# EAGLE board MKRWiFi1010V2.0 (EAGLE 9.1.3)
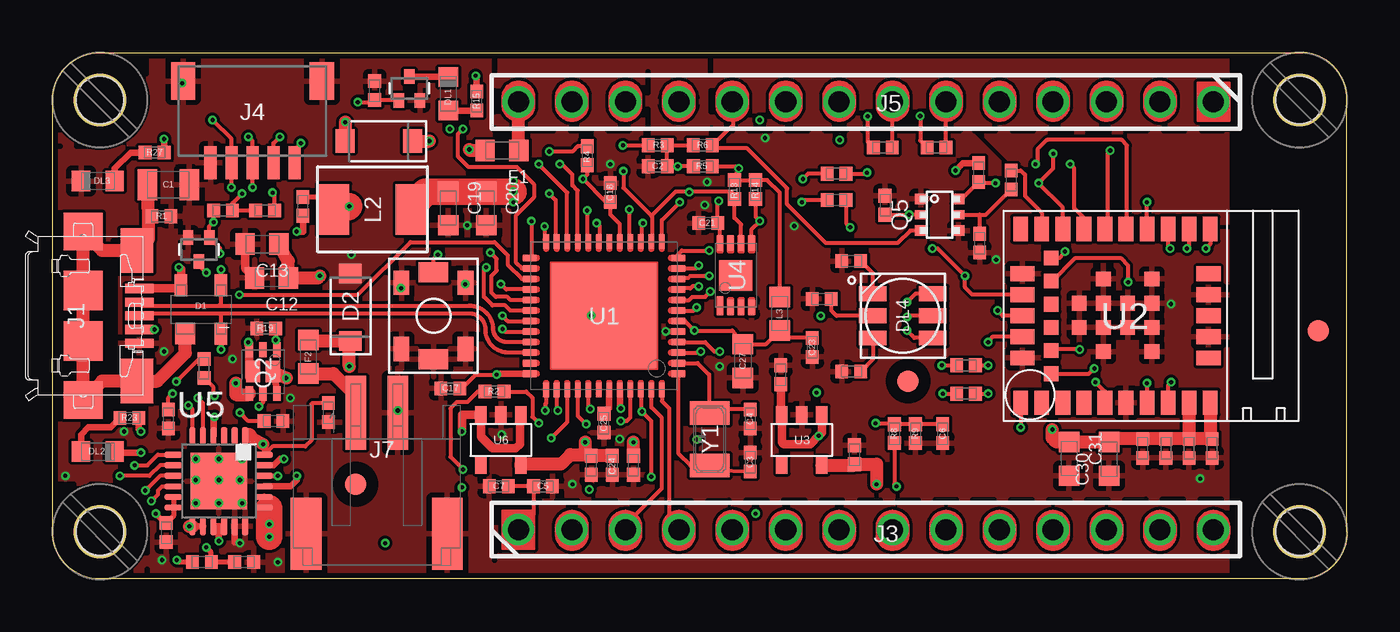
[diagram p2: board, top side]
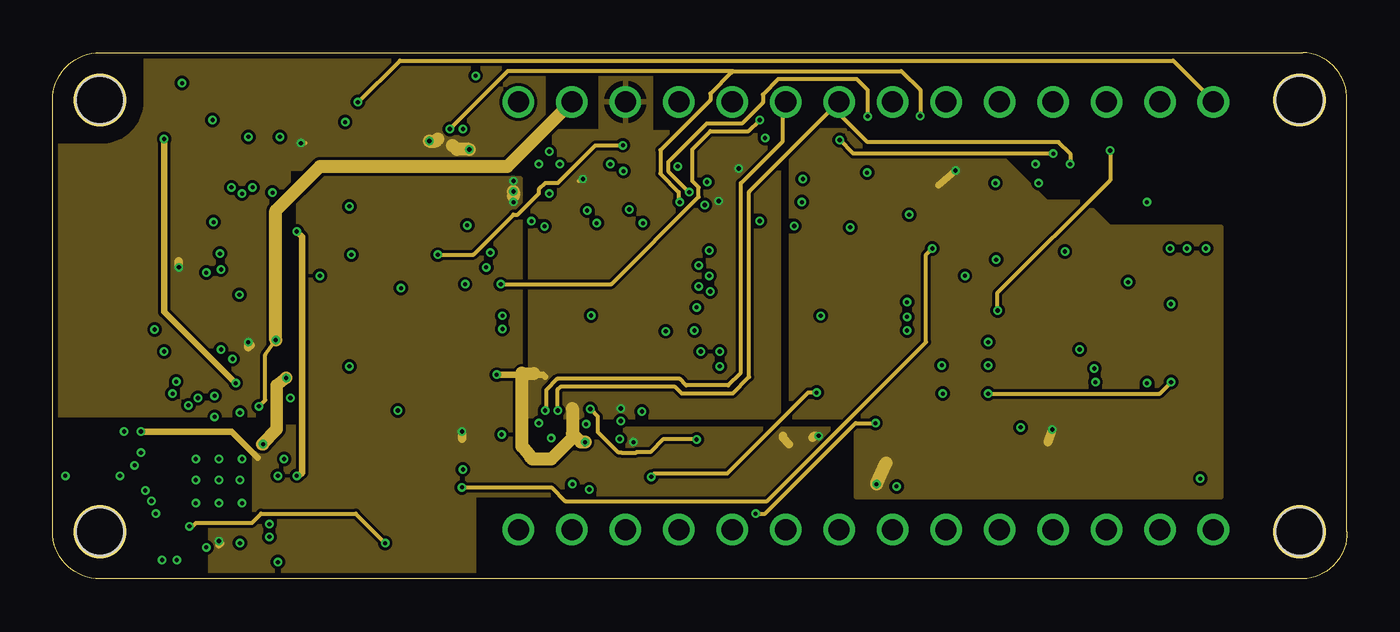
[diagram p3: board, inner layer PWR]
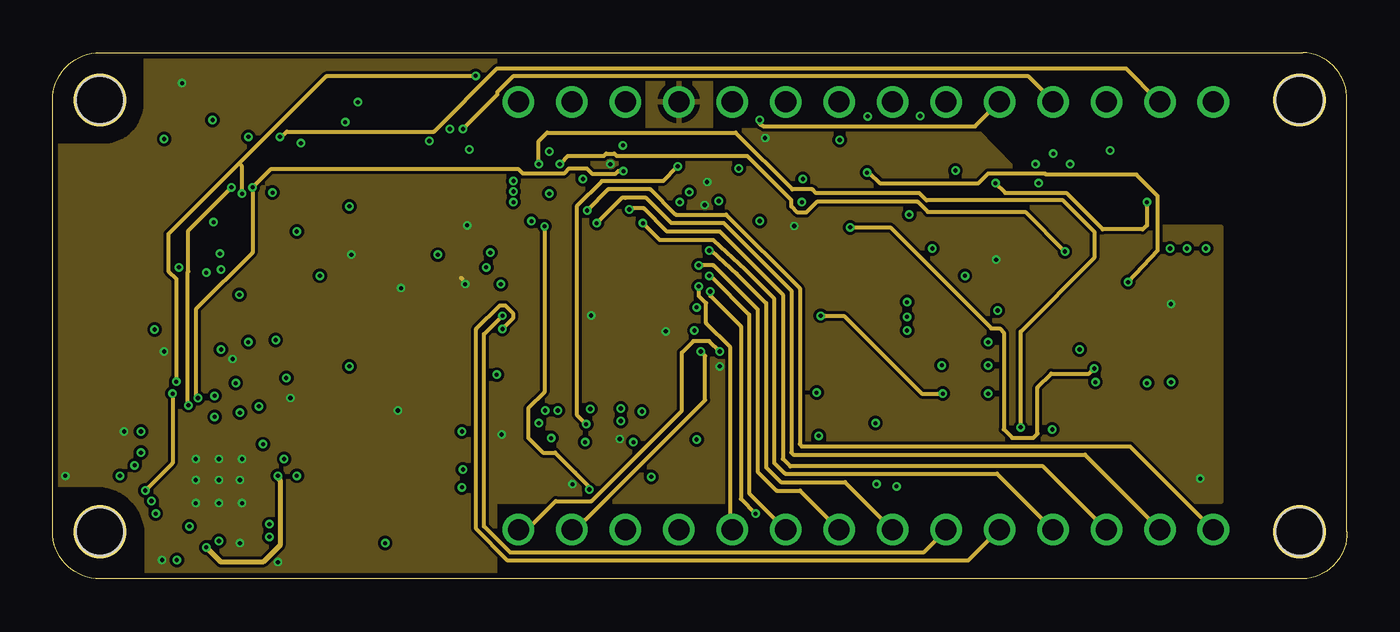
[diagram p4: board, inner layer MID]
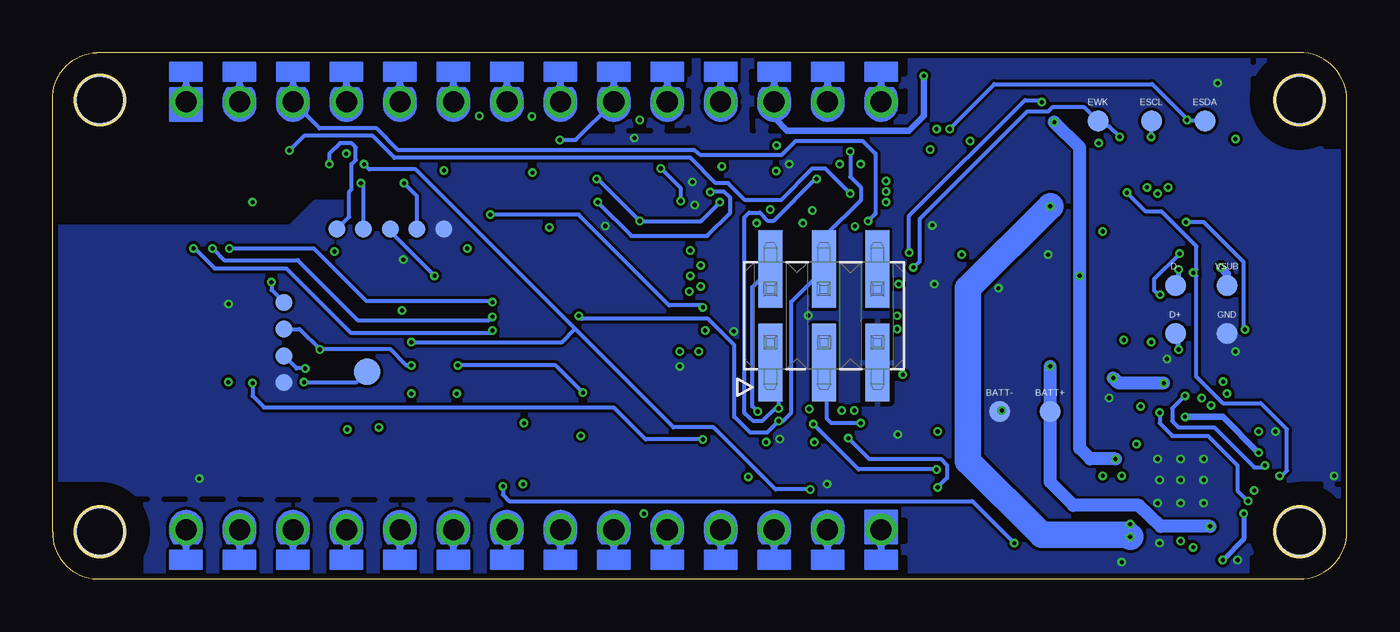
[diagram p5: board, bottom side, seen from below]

Size 61.5 x 25 mm. Coordinates in mm from the lower left corner, seen from the top.
Outline: 0,2.25 0,22.75 arc-90 2.25,25 59.4,25 arc-90 61.5,22.75 61.5,2.25 arc-90 59.4,0 2.25,0 arc-90 0,2.25
Copper layers (1*2*15*16): Top 0.035mm / dielectric 0.2mm / PWR 0.0175mm / dielectric 0.3mm / MID 0.0175mm / dielectric 0.2mm / Bottom 0.035mm
Design rules "B&B_4layers *": minimum track width 6mil, minimum drill 0.195mm, track to track 5.5mil, track to pad 5.5mil, pad to pad 5mil, via to via 5mil, smd to smd 0mil, copper to edge 10mil, drill to drill 8mil, minimum pad ring 6mil, minimum via ring 4mil, stop-mask expansion 4mil, vias tented up to drill 25mil, thermal gap 10mil
Net classes: 0 default: width 0.19 mm, drill 0.19 mm; 1 usb: width 0.19 mm, drill 0.19 mm, clearance 0.127 mm
Holes 2.25 mm at 2.25,2.25 59.25,2.25 59.25,22.75 2.25,22.75
tRestrict: area 0,0 to 4.5,4.5; area 0,20.5 to 4.5,25; area 57,20.5 to 61.5,25; area 57,0 to 61.5,4.5; 119 lines
bRestrict: area 0,0 to 4.5,4.5; area 0,20.5 to 4.5,25; area 57,0 to 61.5,4.5; area 57,20.5 to 61.5,25; 119 lines

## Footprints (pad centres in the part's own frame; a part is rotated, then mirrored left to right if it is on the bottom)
TP-1.00MM = smd 1 x 1 bottom: X 0,0
0805-R2013X50N = smd 0.95 x 1.45: 1 -1,0; 2 1,0
0402-1005X55N = smd 0.62 x 0.62: 1 -0.45,0; 2 0.45,0
0603-1608X90N = smd 0.95 x 1: 1 -0.8,0; 2 0.8,0
SOT190P230X110-4N = smd 1 x 1: 1 -1.15,0.75 | smd 1 x 0.6: 2 -1.15,-0.95; 3 1.15,-0.95; 4 1.15,0.95
SODFL3517X110N = smd 0.91 x 1.07: A 1.605,0; C -1.605,0
LEDC1608X80N-AK = smd 0.9 x 0.95: A 0.8,0; C -0.8,0
RGBLED = smd 1.3 x 0.7: 1 -1.425,1.05; 2 -1.425,0; 3 -1.425,-1.05; 4 1.425,-1.05; 5 1.425,0; 6 1.425,1.05
FD-1-1.5 = smd 1.016 x 1.016: P$1 0,0
TP-0.8MM = smd 0.8 x 0.8 bottom: X 0,0
ZX62-AB-5PA = smd 0.4 x 1.35: 1 -1.3,3.025; 2 -0.65,3.025; 3 0,3.025; 4 0.65,3.025; 5 1.3,3.025 | smd 2.1 x 1.6: 6 3.1,2.9; 11 -3.1,2.9 | smd 1.8 x 1.9: 7 4,0.35; 10 -4,0.35 | smd 1.9 x 1.9: 8 1.2,0.35; 9 -1.2,0.35
2X3_SMT = smd 1.143 x 3.683: 1 -2.54,-2.223; 2 -2.54,2.223; 3 0,-2.223; 4 0,2.223; 5 2.54,-2.223; 6 2.54,2.223
1X14_SMD_TH = drill 1: 1 0,0; 2 2.54,0; 3 5.08,0; 4 7.62,0; 5 10.16,0; 6 12.7,0; 7 15.24,0; 8 17.78,0; 9 20.32,0; 10 22.86,0; 11 25.4,0; 12 27.94,0; 13 30.48,0; 14 33.02,0
SM05B-SRSS-TB = smd 0.6 x 1.55: 1 -2,2.425; 2 -1,2.425; 3 0,2.425; 4 1,2.425; 5 2,2.425 | smd 1.2 x 1.8: SH1 -3.3,-1.45; SH2 3.3,-1.45
JST-S2B-PH-SM4-TB = smd 1 x 3.5: 1 -1,2.95; 2 1,2.95 | smd 1.5 x 3.4: 3 3.35,-2.8; 4 -3.35,-2.8
SRP4020 = smd 1.5 x 2.4: 1 -1.85,0; 2 1.85,0
TP-1.27MM = smd 1.27 x 1.27 bottom: X 0,0
C&K_PTS820_NO_HOLES = smd 1.15 x 0.75: 1 -1.575,1.525; 2 -1.575,-1.525; 3 1.575,1.525; 4 1.575,-1.525 | smd 0.95 x 1.4: 5 -2.075,0; 6 2.075,0
SOTFL50P160X78-3 = smd 0.5 x 0.66: D 0,0.57; G -0.5,-0.57; S 0.5,-0.57
SON65P205X205X75-8N-MWSD = smd 0.67 x 0.37: A 1.04,-0.65; D 1.04,0.65; G -1.04,0; K -1.04,-0.65; NC 1.04,0; S -1.04,0.65 | smd 1 x 0.7: D2 0,0.467; K2 0,-0.467
SOT363 = smd 0.6 x 0.5: 1 -0.9,0.75; 3 -0.9,-0.75; 4 0.9,-0.75; 6 0.9,0.75 | smd 0.6 x 0.4: 2 -0.9,0; 5 0.9,0
QFN50P700X700X90-49XN-EPSQ515 = smd 0.65 x 0.28: 1 -3.525,2.75; 2 -3.525,2.25; 3 -3.525,1.75; 4 -3.525,1.25; 5 -3.525,0.75; 6 -3.525,0.25; 7 -3.525,-0.25; 8 -3.525,-0.75; 9 -3.525,-1.25; 10 -3.525,-1.75; 11 -3.525,-2.25; 12 -3.525,-2.75; 25 3.525,-2.75; 26 3.525,-2.25; 27 3.525,-1.75; 28 3.525,-1.25; 29 3.525,-0.75; 30 3.525,-0.25; 31 3.525,0.25; 32 3.525,0.75; 33 3.525,1.25; 34 3.525,1.75; 35 3.525,2.25; 36 3.525,2.75 | smd 0.28 x 0.65: 13 -2.75,-3.525; 14 -2.25,-3.525; 15 -1.75,-3.525; 16 -1.25,-3.525; 17 -0.75,-3.525; 18 -0.25,-3.525; 19 0.25,-3.525; 20 0.75,-3.525; 21 1.25,-3.525; 22 1.75,-3.525; 23 2.25,-3.525; 24 2.75,-3.525; 37 2.75,3.525; 38 2.25,3.525; 39 1.75,3.525; 40 1.25,3.525; 41 0.75,3.525; 42 0.25,3.525; 43 -0.25,3.525; 44 -0.75,3.525; 45 -1.25,3.525; 46 -1.75,3.525; 47 -2.25,3.525; 48 -2.75,3.525 | smd 5 x 5: 49 0,0
NINA-W1X = smd 0.7 x 1.15: 1 4.95,4.125; 2 3.95,4.125; 3 2.95,4.125; 4 1.95,4.125; 5 0.95,4.125; 6 -0.05,4.125; 7 -1.05,4.125; 8 -2.05,4.125; 9 -3.05,4.125; 10 -4.05,4.125; 16 -4.05,-4.125; 17 -3.05,-4.125; 18 -2.05,-4.125; 19 -1.05,-4.125; 20 -0.05,-4.125; 21 0.95,-4.125; 22 1.95,-4.125; 23 2.95,-4.125; 24 3.95,-4.125; 25 4.95,-4.125 | smd 1.15 x 0.7: 11 -3.975,2; 12 -3.975,1; 13 -3.975,0; 14 -3.975,-1; 15 -3.975,-2; 26 4.875,-2; 27 4.875,-1; 28 4.875,0; 29 4.875,1; 30 4.875,2 | smd 0.7 x 0.7: 31 3.5,2.75; 32 3.5,1.65; 33 3.5,0.55; 34 3.5,-0.55; 35 3.5,-1.65; 36 3.5,-2.75; GND@1 -1.28,1.7; GND@2 -1.28,0.55; GND@3 -1.28,-0.6; GND@4 -1.28,-1.75; GND@5 -0.13,0.55; GND@6 -0.13,-0.6; GND@7 1.02,1.7; GND@8 1.02,0.55; GND@9 1.02,-0.6; GND@10 1.02,-1.75; GND@11 2.17,0.55; GND@12 2.17,-0.6
SOT25 = smd 0.55 x 0.8: 1 0.95,1.2; 2 0,1.2; 3 -0.95,1.2; 4 -0.95,-1.2; 5 0.95,-1.2
SON50P300X200X60-9N-EP160X140 = smd 0.85 x 0.3: 1 -1.45,0.75 | smd 0.7 x 0.3: 2 -1.525,0.25; 3 -1.525,-0.25; 4 -1.525,-0.75; 5 1.525,-0.75; 6 1.525,-0.25; 7 1.525,0.25; 8 1.525,0.75 | smd 1.4 x 1.6: 9 0,0
QFN24 = smd 0.3 x 0.85: 1 1.25,2.155; 2 0.75,2.155; 3 0.25,2.155; 4 -0.25,2.155; 5 -0.75,2.155; 6 -1.25,2.155; 13 -1.25,-2.155; 14 -0.75,-2.155; 15 -0.25,-2.155; 16 0.25,-2.155; 17 0.75,-2.155; 18 1.25,-2.155 | smd 0.85 x 0.3: 7 -2.155,1.25; 8 -2.155,0.75; 9 -2.155,0.25; 10 -2.155,-0.25; 11 -2.155,-0.75; 12 -2.155,-1.25; 19 2.155,-1.25; 20 2.155,-0.75; 21 2.155,-0.25; 22 2.155,0.25; 23 2.155,0.75; 24 2.155,1.25 | smd 2.7 x 2.7: 25 0,0
ABS07 = smd 1.1 x 1.9: 1 -1.25,0; 2 1.25,0

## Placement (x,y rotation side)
BATT+  DNP  [TP-1.00MM]  14.1,7.95 0 top
BATT-  DNP  [TP-1.00MM]  16.5,7.95 0 top
C1  4n7  [0805-R2013X50N]  5.5,18.73 0 top
C2  100n  [0402-1005X55N]  28.75,19.6 180 top
C3  20p  [0402-1005X55N]  33.15,5.55 270 top
C4  20p  [0402-1005X55N]  33.15,7.6 90 top
C5  4u7  [0402-1005X55N]  23.3,4.4 0 top
C6  100n  [0402-1005X55N]  42.3,6.9 270 top
C7  100n  [0402-1005X55N]  21.2,4.4 180 top
C8  100n  [0402-1005X55N]  55.1,6.2 270 top
C9  100n  [0402-1005X55N]  54,6.2 90 top
C12  10u  [0603-1608X90N]  10.4,14.3 180 top
C13  10u  [0603-1608X90N]  9.95,15.9 180 top
C14  1u  [0402-1005X55N]  13.1,7.9 270 top
C15  47n  [0402-1005X55N]  11.9,17.7 90 top
C16  4u7  [0402-1005X55N]  9.1,0.8 0 top
C17  100n  [0402-1005X55N]  18.9,9.05 180 top
C18  100n  [0402-1005X55N]  26.5,18.35 90 top
C19  10u  [0603-1608X90N]  18.8,17.6 270 top
C20  10u  [0603-1608X90N]  20.6,17.6 270 top
C21  100n  [0402-1005X55N]  31.15,16.9 180 top
C22  1u  [0402-1005X55N]  27.6,5.4 270 top
C23  100n  [0402-1005X55N]  36.1,11 270 top
C24  100n  [0402-1005X55N]  26.6,5.4 270 top
C25  1u  [0402-1005X55N]  26.2,7.4 270 top
C26  1u  [0402-1005X55N]  25.6,5.4 270 top
C27  4u7  [0603-1608X90N]  32.8,10.35 270 top
C28  DNP  [0402-1005X55N]  52.9,6.2 90 top
C29  DNP  [0402-1005X55N]  51.8,6.2 270 top
C30  DNP  [0603-1608X90N]  50.2,5.7 90 top
C31  DNP  [0603-1608X90N]  48.3,5.7 270 top
C32  1u  [0402-1005X55N]  34.6,9.7 90 top
C33  1u  [0402-1005X55N]  38.1,5.9 90 top
D1  PRTR5V  [SOT190P230X110-4N]  7.05,12.8 90 top
D2  PMEG6020  [SODFL3517X110N]  14.15,12.9 90 top
D3  PMEG6020  [SODFL3517X110N]  15.5,20.8 180 top
D+  DNP  [TP-1.00MM]  8.15,11.65 0 top
D-  DNP  [TP-1.00MM]  8.15,13.95 0 top
DL1  YELLOW  [LEDC1608X80N-AK]  18.8,23.05 270 top
DL2  ORANGE  [LEDC1608X80N-AK]  2.15,6.05 180 top
DL3  GREEN  [LEDC1608X80N-AK]  2.15,18.9 0 top
DL4  RGB  [RGBLED]  40.4,12.5 180 top
ESCL  DNP  [TP-1.00MM]  9.29,21.75 0 top
ESDA  DNP  [TP-1.00MM]  6.75,21.75 0 top
EWK  DNP  [TP-1.00MM]  11.83,21.75 0 top
F1  MFFSMF050  [0603-1608X90N]  21.35,20.35 180 top
F2  MFFSMF050  [0603-1608X90N]  12.15,10.55 90 top
FD1  DNP  [FD-1-1.5]  14.4,4.5 0 top
FD2  DNP  [FD-1-1.5]  60.15,11.8 0 top
FD3  DNP  [FD-1-1.5]  40.65,9.4 0 top
FRAME1  DNP  [FRAME]  not placed on the board
FRAME2  [FRAME-NO-BAN-FRAMEONLY]  not placed on the board
GND  DNP  [TP-1.00MM]  5.7,11.65 0 top
GPIO0  DNP  [TP-0.8MM]  45.46,16.62 0 top
J1  -  [ZX62-AB-5PA]  1.1,12.5 270 top
J2  DNP  [2X3_SMT]  24.85,12.5 0 bottom
J3  -  [1X14_SMD_TH]  22.13,2.34 0 top
J4  -  [SM05B-SRSS-TB]  9.5,22.2 180 top
J5  -  [1X14_SMD_TH]  55.15,22.66 180 top
J7  -  [JST-S2B-PH-SM4-TB]  15.4,4.95 0 top
JCLK  DNP  [TP-0.8MM]  50.5,13.13 0 top
JGND  DNP  [TP-0.8MM]  50.5,9.32 0 top
JTDO  DNP  [TP-0.8MM]  50.5,11.87 0 top
JTMS  DNP  [TP-0.8MM]  50.5,10.6 0 top
L2  2u2  [SRP4020]  15.2,17.55 0 top
L3  BLM18PG471  [0603-1608X90N]  34.55,12.6 270 top
LPO_IN  DNP  [TP-1.27MM]  46.55,9.85 0 top
PB1  PTS820  [C&K_PTS820_NO_HOLES]  18.1,12.5 90 top
PGND  DNP  [TP-0.8MM]  42.92,16.62 0 top
Q1  2N7002  [SOTFL50P160X78-3]  16.95,23.3 0 top
Q2  SIA817  [SON65P205X205X75-8N-MWSD]  10,9.85 90 top
Q3  2N7002  [SOTFL50P160X78-3]  6.95,15.65 180 top
Q5  BSS138PS  [SOT363]  42.15,17.3 0 top
R1  1M  [0402-1005X55N]  5.17,17.23 180 top
R2  39R  [0402-1005X55N]  21,8.9 180 top
R3  330R  [0402-1005X55N]  28.75,20.6 0 top
R4  1k  [0402-1005X55N]  25.4,20.1 270 top
R5  10k  [0402-1005X55N]  30.9,19.6 0 top
R6  330R  [0402-1005X55N]  30.89,20.6 0 top
R7  10k  [0402-1005X55N]  44,19.3 90 top
R8  330k  [0402-1005X55N]  40,6.9 270 top
R9  1M2  [0402-1005X55N]  41,6.9 90 top
R10  100k  [0402-1005X55N]  39.55,17.75 90 top
R11  100k  [0402-1005X55N]  44.05,15.95 270 top
R12  0R  [0402-1005X55N]  43.4,8.8 0 top
R13  4k7  [0402-1005X55N]  32.4,18.5 90 top
R14  4k7  [0402-1005X55N]  33.4,18.5 90 top
R15  330R  [0402-1005X55N]  20.15,22.7 270 top
R16  100k  [0402-1005X55N]  15.3,23.2 270 top
R17  0R  [0402-1005X55N]  45.55,18.95 270 top
R18  0R  [0402-1005X55N]  37.25,19.25 180 top
R19  100k  [0402-1005X55N]  10.15,11.9 0 top
R20  0R  [0402-1005X55N]  37.25,18 180 top
R21  10k  [0402-1005X55N]  8.1,17.5 180 top
R22  0R  [0402-1005X55N]  43.4,10.15 0 top
R23  330R  [0402-1005X55N]  3.65,7.65 0 top
R24  10k  [0402-1005X55N]  7.2,10 270 top
R25  10k  [0402-1005X55N]  5.5,7.6 90 top
R26  10k  [0402-1005X55N]  10.1,17.5 0 top
R27  390R  [0402-1005X55N]  4.85,20.25 0 top
R28  330R  [0402-1005X55N]  10.5,7.5 0 top
R29  10k  [0402-1005X55N]  5.4,2.2 90 top
R30  5k49  [0402-1005X55N]  7.1,0.8 180 top
R31  0R  [0402-1005X55N]  42,20.5 180 top
R32  0R  [0402-1005X55N]  39.45,20.5 180 top
R34  330R  [0402-1005X55N]  36.55,13.3 0 top
R35  330R  [0402-1005X55N]  37.95,9.85 0 top
R36  330R  [0402-1005X55N]  37.95,15.1 0 top
RST  DNP  [TP-0.8MM]  44.19,16.62 0 top
RXD  DNP  [TP-0.8MM]  46.73,16.62 0 top
TXD  DNP  [TP-0.8MM]  48,16.62 0 top
U1  D21G18  [QFN50P700X700X90-49XN-EPSQ515]  26.2,12.5 180 top
U2  NINA-W102  [NINA-W1X]  50.95,12.5 180 top
U3  AP2112K-3.3  [SOT25]  35.6,6.6 0 top
U4  ECC508  [SON50P300X200X60-9N-EP160X140]  32.46,14.43 90 top
U5  BQ24195L  [QFN24]  7.9,4.65 0 top
U6  AP2112K-3.3  [SOT25]  21.3,6.6 0 top
U$5  [MH_RND_F_2.2MM_NM]  2.25,2.25 90 top
U$6  [MH_RND_F_2.2MM_NM]  2.25,22.75 90 top
U$7  [MH_RND_F_2.2MM_NM]  59.25,22.75 90 top
U$8  [MH_RND_F_2.2MM_NM]  59.25,2.25 90 top
VSUB  DNP  [TP-1.00MM]  5.7,13.95 0 top
Y1  32768Hz  [ABS07]  31.23,6.64 270 top

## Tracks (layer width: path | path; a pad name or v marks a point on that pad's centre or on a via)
+3V3  (via drill 0.2)
  Top 0.19: v5.88,9.38 6.88,10.38 7.12,10.38 R24.1
  Top 0.2: U4.8 31.71,16.74 C21.1 31.6,17.9 v31.65,17.95 | R5.2 32.5,19.6 v32.6,19.5 R13.2 R14.2 33.95,18.95 34.55,18.35 L3.1 | U1.17 26.95,16.85 26.5,17.3 C18.1 26.3,17.9 v25.2,19 25.4,19.2 R4.2 | C17.1 19.4,9 20.1,9.7 v21.1,9.7 | R26.1 R21.1 8.55,17.85 v9,18.3
  Top 0.305: U1.44 26.95,8.15 v27,8.1 | U1.36 21.15,9.75 v21.1,9.7 | R15.1 20.15,23.85 v20.1,23.9
  Top 0.61: 25.1,5.9 24.6,5.9 24.15,5.45 22.25,5.45 U6.5 | 25.1,5.9 25.55,5.9 C26.1 C24.1 | v25.3,6.5 25.3,6.1 25.1,5.9
  PWR 0.2: v25.2,19 25.1,19 25,18.9
  PWR 0.305: v21.1,9.7 23.3,9.7 23.4,9.6
  PWR 0.61: v25.3,6.5 25.1,6.5 24.8,6.8 | 24.8,6.8 24.7,6.9 24.7,8.1 | 22.88,9.75 22.3,9.78 22.3,6.3 22.7,5.8 22.8,5.7 23.7,5.7 24.8,6.8
  MID 0.19: v5.88,9.38 5.88,14.25 5.5,14.62 5.5,16.38 8.86,19.74 13,23.88 20,23.88 v20.1,23.9
  MID 0.2: v9,18.3 9,19.6 8.86,19.74
  Bottom 0.19: 25.25,19 v25.2,19 | 32.62,19.5 v32.6,19.5
  Bottom 0.2: 25.25,19 27.25,17 27.5,17 27.9,17.4 28.4,17.4 28.62,17.18 28.62,7.88 28.6,7.85 28.2,7.5 27.8,7.5 27.15,8.1 v27,8.1 27,9.89 | v31.65,17.95 31.65,18.55 v32.6,19.5
  Bottom 0.305: 27,9.89 J2.1 | v20.1,23.9 20.1,22 20.8,21.3 26.6,21.3 27.2,21.9 27.2,22.64 J5.12
  pour PWR: 26.05,25 26.05,21.25 23.85,21.25 23.85,17.85 23.8,17.8 22.7,17.8 22.7,7.7 34.5,7.7 34.5,21.2 28.4,21.2 28.4,24.95
+3V3D  (via drill 0.2)
  Top 0.305: R7.2 43.25,19.75 v42.9,19.4
  Top 0.406: 50.35,6.65 C30.2 | 55,6.75 C8.1
  Top 0.61: C8.1 C9.2 | C9.2 C28.2 C29.1 50.35,6.65 | C30.2 C31.1 47.7,6.5 47.5,6.7 v47.5,7.1 | U2.10 55,6.75 | U2.9 C9.2 | U3.5 38.05,5.4 C33.1 39.15,5.45 v39.15,4.5
  PWR 0.305: v42.9,19.4 42.2,18.8 42.1,18.7
  PWR 0.406: v47.5,7.1 47.3,6.5
  PWR 0.61: v39.15,4.5 39.6,5.5
  pour PWR: 35.1,21.3 35.1,7.7 38.2,7.7 38.2,3.9 55.5,3.9 55.5,16.7 50.2,16.7 49,17.9 47.2,17.9 43.8,21.3
+3V8  (via drill 0.2)
  Top 0.305: U5.15 U5.16 8.1,2.5 7.9,2.3 v7.9,1.8 | R23.2 4.1,7.1 v4.2,7
  Top 0.406: v19.45,7 19.45,7.8 U6.3 20.35,6.75 20.9,6.2 22,6.2 22.2,6.4 22.2,7.75 U6.1 | U3.1 36.55,6.95 v36.4,6.8 36,6.4 34.75,6.4 34.65,6.5 U3.3 34.6,7.85 C32.1
  Top 0.61: C22.1 v27.6,6.5
  Top 1.27: L2.2 17.7,18.4 C19.1 C20.1 v21.9,18.4
  PWR 0.305: v7.9,1.8 7.9,1.6 8,1.7 | v4.2,7 8.5,7 9.75,5.75
  PWR 0.406: v19.45,7 19.45,6.65 | 34.7,6.8 34.7,6.7 35,6.4 | v36.4,6.8 36.2,6.8 36.1,6.7
  PWR 0.61: v21.9,18.4 21.9,18.2
  other vias: 21.9,18.9 21.9,17.9
  pour PWR: 9.6,7.2 11.7,7.2 11.7,19 22.2,19 22.2,7.1 37.6,7.1 37.6,4 20,4 20,0 7.5,0 7.5,2.9 9.6,2.9
+5V  (via drill 0.2)
  Top 0.2: J4.1 11.5,20.4 v11.8,20.7
  Top 0.406: J1.1 5.95,13.8 D1.4 6.1,14.7 v6,14.8 | Q2.D2 9.35,9.58 Q2.D 9.35,11 v9.3,11.25
  Top 0.61: F1.2 19.85,20.35 v19.8,20.4 | D3.C v17.9,20.8
  PWR 0.2: v11.8,20.7 12,20.7
  PWR 0.406: v6,14.8 6,15.1 | v9.3,11.25 9.3,11 9.4,11.1
  PWR 0.61: v19.8,20.4 19.2,20.4 19,20.6 | v17.9,20.8 18.2,20.8 18.3,20.9
  Bottom 0.406: VSUB.X 5.7,14.5 v6,14.8
  pour PWR: 23.3,25 4.45,25 4.45,22.7 arc-90 2.3,20.55 0,20.55 0,7.8 11.2,7.8 11.2,19.5 23.3,19.5
GND  (via drill 0.2)
  Top 0.2: PB1.4 19.62,14.03 v19.6,14
  Top 0.305: U5.17 8.65,1.75 v8.9,1.7
  Top 0.406: C13.2 9.15,14.75 C12.2
  MID 0.2: v19.6,14 19.6,14.1 19.4,14.3
  other vias: 31.7,10.1 6.8,5.7 7.9,5.7 9,5.7 9,3.6 7.9,3.6 6.8,3.6 6.8,4.7 7.9,4.7 8.9,4.7 5.3,10.8 5.2,0.9 10.7,0.8 24.7,4.5 26.95,6.65 26.5,19.7 8.55,10.45 3.4,7 14.2,15.4 16.55,13.81 19.7,16.8 25.59,12.52 16.4,8 30.98,17.77 29.14,11.77 31.1,18.85 0.6,4.9 6.15,23.55 35.23,16.77 44.84,15.16 53.13,13.06 33.85,20.95 54.53,4.76 11.3,8.6 21.34,6.87
  pour Bottom: 0,0 0,25 43.8,25 43.8,21.2 47.1,17.9 49,17.9 50.2,16.7 61.5,16.7 61.5,0
  pour Top: 0,-0.1 0,24.9 28.5,25 55.8,25.1 55.8,0.1
  pour MID: 0,20.55 2.4,20.55 arc90 4.45,22.6 4.45,25 21,25 21,21.3 28.3,21.3 28.3,25 31.25,25 31.25,21.3 43.9,21.3 47.2,17.9 49,17.9 50.2,16.7 55.5,16.7 55.5,3.7 21,3.7 21,0 4.5,0 4.5,2.1 arc90 2.1,4.5 0,4.5
LED_BLUE  (via drill 0.2)
  Top 0.2: DL4.2 40.65,12.5 v40.6,12.45 | U2.17 54,15.8 v53.9,15.7
  Bottom 0.2: 40.7,12.35 v40.6,12.45 40.75,12.3 47,12.3 49.85,15.15 53.35,15.15 v53.9,15.7
LED_GREEN  (via drill 0.2)
  Top 0.2: DL4.1 40.95,11.45 v40.6,11.8 | U2.16 55,15.9 v54.8,15.7
  Bottom 0.2: v40.6,11.8 40.7,11.7 47.35,11.7 50.4,14.75 53.8,14.75 54.75,15.7 v54.8,15.7
LED_RED  (via drill 0.2)
  Top 0.2: 40.59,13.13 v40.6,13.15 41,13.55 DL4.3 | U2.18 53,15.8 v53.1,15.7
  Bottom 0.2: v40.6,13.15 40.65,13.2 46.59,13.2 49.09,15.7 v53.1,15.7
N17658775  (via drill 0.2)
  Top 0.2: PB1.6 18.1,15.2 v18.3,15.4 | v27.1,20.6 R3.1
  PWR 0.2: v27.1,20.6 25.8,20.6 24,18.8 23.4,18.8 23.1,18.5 23.1,18.3 22.1,17.3 21.9,17.3 20,15.4 v18.3,15.4
N17798864
  Top 0.305: DL2.A 1.35,6.85 1.7,7.2 2.75,7.2 R23.1
N17834267
  Top 0.305: 3.05,18.9 DL3.A 2.95,19.5 3.7,20.25 R27.1
N17852357  (via drill 0.2)
  Top 0.2: U1.6 30.05,12.25 v30.5,11.8 32.3,11.8 C27.1 33.9,11.15 L3.2 34.9,11.45 C23.1
N17852431
  Top 0.305: U1.43 26.45,8.1 C25.1
N$1
  Top 0.61: C1.1 4.55,17.15 | 4.55,17.15 4.55,16.15 J1.11 2.35,15.6 J1.10 J1.9 J1.8 J1.7 2.35,9.4 J1.6 4.97,9.4 6.3,10.72 D1.1 | R1.2 4.55,17.15
N$2
  Top 0.61: F1.1 22.15,22.64 J5.14
N$3
  Top 0.61: F2.1 13.35,9.75 14.4,8.7 J7.1
N$4  (via drill 0.2)
  Top 0.2: R2.1 22.5,8.9 22.8,8.6 22.8,7.7 v23.1,7.4
  Bottom 0.2: J2.3 24.7,10.13 24.7,7.6 24.5,7.4 v23.1,7.4
N$5
  Top 0.2: R32.1 39.9,22.64 J5.7
N$6  (via drill 0.2)
  Top 0.2: U1.8 30.25,13.25 30.4,13.4 31,13.4 v31.25,13.65 | C6.1 R9.2 R8.1 39.95,7.4 v39.1,7.4
  PWR 0.2: v33.4,3.1 33.85,3.1 38.15,7.4 v39.1,7.4
  MID 0.2: v31.25,13.65 31.25,13.45 32.7,12 32.7,3.8 v33.4,3.1
N$7
  Top 0.305: DL1.A R15.2
N$8
  Top 0.2: R31.1 J5.6
N$9  (via drill 0.2)
  Top 0.2: U2.19 v52,17.9 | 43.92,18.77 R7.1 | v44.8,18.8 44.05,18.8 R7.1 | Q5.6 43.2,18.05 R7.1
  MID 0.2: v52,17.9 52,16.8 51.8,16.6 49.9,16.6 48.16,18.34 45.26,18.34 v44.8,18.8
  Bottom 0.2: RST.X 44.19,18.19 v44.8,18.8
N$10
  Top 0.305: DL1.C 16.97,23.85 Q1.D
N$11  (via drill 0.2)
  Top 0.2: U2.35 47.5,14.15 48.6,15.25 50.75,15.25 51.1,14.9 v51.1,14.1 | R18.1 38.65,19.25 v38.7,19.3
  MID 0.2: v38.7,19.3 38.8,19.3 39.3,18.8 44,18.8 44.45,19.25 47.15,19.25 47.2,19.2 51.5,19.2 52.5,18.2 52.5,15.6 v51.1,14.1
  Bottom 0.2: v51.1,14.1 51.1,13.73 JCLK.X
N$12  (via drill 0.2)
  Top 0.2: U2.31 49.25,9.75 v49.5,10 | R20.1 37.7,16.9 v37.9,16.7
  MID 0.2: v37.9,16.7 39.8,16.7 44.6,11.9 45,11.9 45.2,11.7 45.2,7.1 45.6,6.7 46.6,6.7 46.8,6.9 46.8,9.1 U2.31 49.25,9.75 v49.5,10
  Bottom 0.2: v49.5,10 49.91,10 JTMS.X
N$13
  Top 0.2: U2.24 47,17.4 46.2,18.2 46.2,19.2 46,19.4 R17.1
N$14
  Top 0.2: DL4.5 37.25,12.5 37,12.75 R34.2
N$15  (via drill 0.2)
  Top 0.24: C15.2 13.15,18.15 L2.1
  Top 0.305: v10.3,2.6 10.3,3.35 10.24,3.4 U5.19 U5.20
  Top 1.27: L2.1 14.05,17.65 v14.1,17.7 | v10.3,2 10.3,3.35
  Bottom 1.27: v10.3,2 10.4,2.1 14.5,2.1 18,5.6 18,13.8 v14.1,17.7
N$16
  Top 0.2: DL4.6 38.98,10.43 R35.2
N$17  (via drill 0.2)
  Top 0.19: 10.1,6.2 v10,6.4
  Top 0.2: 10.1,6.1 10.1,5.95 U5.24 10.46,6.3 12,6.3 12.3,6.6 12.3,8.3 12.35,8.35 C14.1 | U5.1 9.29,6.8
  Top 0.305: Q2.K 10.65,9.12 Q2.K2 | R27.2 v5.3,20.9 | 10.1,6.1 10.1,6.2
  Top 0.605: 9.39,6.8 9.29,6.8 v10,6.4
  Top 0.61: 9.35,6.85 9.39,6.8 9.4,6.8 | Q2.K2 v11.1,9.55 | v8.7,9.3 8.7,8.75 9.31,8.75 Q2.S
  PWR 0.305: v5.3,20.9 5.3,12.7 v8.7,9.3
  PWR 0.605: v10,6.4 9.95,6.4 10.65,7.1 10.65,9.2 v11.1,9.55
  Bottom 0.61: v8.7,9.3 10.85,9.3 v11.1,9.55
N$18  (via drill 0.2)
  Top 0.305: U5.21 11.3,4.4 11.6,4.7 v11.6,4.9 | v11.6,16.5 11.9,16.5 C15.1
  PWR 0.305: v11.6,4.9 11.7,4.9 11.85,5.05 11.85,16.25 v11.6,16.5
N$19  (via drill 0.2)
  Top 0.2: U5.10 5.2,4.4 5,4.2 5,4 v4.7,3.7 | R28.1 9.3,7.5 v8.9,7.9
  Bottom 0.2: v8.9,7.9 8.9,7.4 8.3,6.8 6.6,6.8 5.2,5.4 5.2,4.2 v4.7,3.7
N$20
  Top 0.2: DL4.4 38.98,14.53 R36.2
N$21  (via drill 0.2)
  Top 0.24: C16.1 R30.1 7.5,0.85 7.5,1.3 v7.3,1.5 | U5.22 v10.7,4.9
  MID 0.24: v10.7,4.9 10.7,4.8 10.8,4.7 10.8,1.6 10,0.8 8,0.8 v7.3,1.5
N$22  (via drill 0.2)
  Top 0.2: U5.8 5.1,5.4 4.6,4.9 v3.2,4.9 | R26.2 10.55,18.3 v10.45,18.35 | Q3.D 6.95,14.9 v7.3,14.55
  Bottom 0.2: v3.2,4.9 3.1,4.9 2.85,5.15 2.85,7.1 4.1,8.35 5.9,8.35 7.15,9.6 7.15,14.4 v7.3,14.55 7.15,14.7 7.15,15.8 8.8,17.45 9.55,17.45 v10.45,18.35
N$23  (via drill 0.2)
  Top 0.24: U5.11 U5.12 5.75,3 R29.2 5.35,2.65 v4.9,3.1 | R30.2 6,0.8 v5.9,0.9
  Bottom 0.24: v4.9,3.1 4.9,1.9 v5.9,0.9
N$24  (via drill 0.2)
  Top 0.2: R25.2 5.5,8.6 v5.7,8.8 | U5.9 5.1,4.9 v4.4,4.2
  MID 0.2: v5.7,8.8 5.7,5.5 v4.4,4.2
N$25  (via drill 0.2)
  Top 0.2: U2.5 50,8.9 v49.55,9.35
  Bottom 0.2: v49.55,9.35 47.05,9.35 LPO_IN.X
N$26  (via drill 0.2)
  Top 0.2: v48.8,10.9 47.5,10.9 U2.32 | R22.2 v44.45,10.15
  Bottom 0.2: JTDO.X 49.77,11.87 v48.8,10.9 45.45,10.9 44.7,10.15 v44.45,10.15
N$27  (via drill 0.2)
  Top 0.2: R12.2 v44.45,8.8 | v53.15,9.35 53,9.2 U2.8
  PWR 0.2: v44.45,8.8 52.6,8.8 v53.15,9.35
N$28
  Top 0.2: Q5.5 44.05,17.3 | 44.05,17.3 44.35,17.3 R17.2 | R11.1 44.05,17.3
PA00_XIN32
  Top 0.2: U1.1 29.73,5.97 30.3,5.4 31.21,5.4 Y1.2 31.46,5.15 C3.2
PA01_XOUT32
  Top 0.2: U1.2 30.65,10.25 31.2,9.7 31.2,8.61 Y1.1 31.39,8.05 C4.2
PA02_AIN0  (via drill 0.2)
  Top 0.2: U1.3 30.75,10.75 v30.8,10.8
  MID 0.2: J3.2 25.14,2.8 25.3,2.8 31,8.5 31,10.6 v30.8,10.8
PA03_VREFA  (via drill 0.2)
  Top 0.2: U1.4 31,11.25 31.45,10.8 v31.7,10.8 | C7.1 C5.1 22.85,3.06 J3.1
  MID 0.2: v31.7,10.8 31.2,11.3 30.45,11.3 29.9,10.75 29.9,8 25.6,3.7 23.9,3.7 22.61,2.4 22.2,2.4 J3.1
PA04_AIN4  (via drill 0.2)
  Top 0.2: v30.7,13.9 30.4,13.9 30.3,13.8 29.77,13.8 U1.9
  MID 0.2: J3.5 32.3,2.4 32.2,2.4 32.2,11 31.05,12.15 31.05,13.1 30.7,13.45 v30.7,13.9
PA05_AIN5  (via drill 0.2)
  Top 0.2: U1.10 29.77,14.3 30.2,14.3 30.3,14.4 v31.2,14.4
  MID 0.2: v31.2,14.4 31.3,14.4 31.3,14.35 33.1,12.55 33.1,4.08 J3.6
PA06_AIN6  (via drill 0.2)
  Top 0.2: U1.11 30.55,14.75 v30.7,14.9
  MID 0.2: v30.7,14.9 31.4,14.9 33.5,12.8 33.5,5.1 34.4,4.2 35.52,4.2 J3.7
PA07_AIN7  (via drill 0.2)
  Top 0.2: U1.12 29.73,15.43 29.9,15.6 v31.2,15.6
  MID 0.2: v31.2,15.6 31.3,15.6 32.5,14.5 33.9,13.1 33.9,5.3 34.6,4.6 37.66,4.6 J3.8
PA08_S0_I2C_SDA  (via drill 0.2)
  Top 0.2: U1.13 28.95,17.05 v29.8,17.9 | 33.61,16.99 v33.6,17 | v7.6,21.8 8.5,20.9 J4.4 v8.5,18.6 | U5.6 6.65,8.05 v6.45,8.25 | U4.5 33.21,16.61 v33.6,17 | R14.1 33.4,17.2 v33.6,17 | R18.2 35.9,19.25 v35.65,19 | v41.23,21.99 41.23,20.82 R31.2
  PWR 0.19: 32.33,24.12 32.26,24.06 | 32.26,24.06 31.25,23.05 31.25,22.75 28.88,20.38 28.88,19.25 29.75,18.38 29.75,18 v29.8,17.9 | v18.88,21.38 21.62,24.12 32.25,24.12 32.26,24.06
  PWR 0.2: 32.33,24.12 40.33,24.12 41.23,23.23 v41.23,21.99
  MID 0.2: v6.45,8.25 6.4,8.3 6.4,14.55 6.45,14.6 6.45,16.55 v8.5,18.6
  Bottom 0.19: v18.88,21.38 16.75,23.5 9.25,23.5 7.62,21.88 v7.6,21.8
  Bottom 0.2: v7.6,21.8 6.8,21.8 ESDA.X | v29.8,17.9 30.7,17 v33.6,17 35.6,19 v35.65,19
PA09_S0_I2C_SCL  (via drill 0.2)
  Top 0.19: v30.25,18.38 30.25,18.4 | v27.12,19.38 27.12,19.25
  Top 0.2: 28.5,16.07 U1.14 28.48,16.02 28.5,16.05 28.5,17.2 28.45,17.25 | 28.45,17.25 29.6,18.4 30.25,18.4 32.25,18.4 R13.1 32.4,17.15 32.71,16.84 U4.6 | v9.3,21 9.5,20.8 J4.3 v9.5,18.6 | U5.5 7.15,8.35 v6.9,8.6 | 27.12,19.25 27.12,18.57 28.45,17.25 | R20.2 35.7,18 v35.6,17.9 | v38.73,21.98 38.73,20.77 R32.2
  PWR 0.19: v30.25,18.38 29.25,19.38 29.25,19.8 31.07,21.62 32.75,21.62 33.75,22.62 33.75,23 34.5,23.75
  PWR 0.2: 34.5,23.75 38.2,23.75 38.73,23.23 v38.73,21.98
  MID 0.19: v27.12,19.38 26.88,19.38 26.75,19.25 25.62,19.25 25.38,19.5 24.55,19.5
  MID 0.2: 24.55,19.5 24.3,19.25 22.35,19.25 22.15,19.45 10.35,19.45 v9.5,18.6 9.5,15.5 6.8,12.8 6.8,8.7 v6.9,8.6
  Bottom 0.2: v9.3,21 ESCL.X | v35.6,17.9 34,16.3 30.4,16.3 29.3,17.4 29.3,18.1 29.6,18.4 30.23,18.4 v30.25,18.38
PA10_TCC0-W2  (via drill 0.2)
  Top 0.2: U1.15 28,16.07 28,16.85 v28.05,16.9
  PWR 0.2: 47.5,2.38 J3.11
  MID 0.2: 47.5,2.38 J3.11 44.88,5 34.8,5 34.3,5.5 34.3,13.3 32.9,14.7 31.4,16.1 28.85,16.1 v28.05,16.9
PA11_TCC0-W3  (via drill 0.2)
  Top 0.2: v27.4,17.55 27.4,16.07 U1.16
  MID 0.2: v27.4,17.55 27.5,17.6 28.1,17.6 29.2,16.5 31.7,16.5 34.7,13.5 34.7,5.7 35.05,5.35 47.06,5.35 J3.12
PA12_S2_TX/MOSI  (via drill 0.2)
  Top 0.2: v24.1,19.7 24.2,19.7 24.7,19.2 24.7,18.7 24.95,18.45 U1.21 | U2.36 47.85,15.25 47.9,15.3 v48.1,15.55
  MID 0.2: v24.1,19.7 24.5,20.1 26.2,20.1 26.3,20.2 26.7,20.2 26.8,20.1 33,20.1 35.1,18 35.1,17.7 35.4,17.4 35.8,17.4 36.31,17.91 41.11,17.91 41.59,17.44 46.21,17.44 v48.1,15.55
PA13_S2_RX/MISO  (via drill 0.2)
  Top 0.2: U1.22 24.45,18.35 v23.1,19.7 | U2.1 v46,7.2
  MID 0.2: v46,7.2 46,11.75 49.5,15.25 49.5,16.5 48.01,17.99 41.52,17.99 41.19,18.32 36.27,18.32 36.1,18.5 35.15,18.5 32.45,21.2 23.5,21.2 23.1,20.8 v23.1,19.7
PA14_S2_RTS/CS  (via drill 0.2)
  Top 0.2: v23.6,18.3 23.9,18 23.9,16.07 U1.23 | U2.28 45.15,12.5 v44.9,12.75 | U2.21 50.15,16.77 50.15,20.25 v50.25,20.35
  PWR 0.2: v44.9,12.75 44.9,13.6 50.25,18.95 v50.25,20.35
  Bottom 0.2: v23.6,18.3 24.8,19.5 25.4,19.5 26.9,18 28.6,18 29.4,18.8 30,18.8 31.2,20 45.25,20 46.3,21.05 49.55,21.05 v50.25,20.35
PA15_S2_CTS/SCK  (via drill 0.2)
  Top 0.19: v23.38,16.75 23.38,16.12 U1.24
  Top 0.2: U2.29 44.65,11.5 v44.45,11.25 | v46.7,19.7 46.8,19.8 46.8,20.4 47.25,20.85 50.8,20.85 51.05,20.6 51.05,16.68 U2.20
  MID 0.19: 24.82,5.05 25.5,4.38 v25.5,4.25
  MID 0.2: v23.38,16.75 23.38,8.88 22.6,8.1 22.6,6.7 23.3,6 23.88,6 24.82,5.05
  Bottom 0.2: v44.45,11.25 37.3,11.25 36.67,11.88 | 36.67,11.88 44.25,19.45 46.45,19.45 v46.7,19.7 | 36.67,11.88 32,7.2 30.1,7.2 27.15,4.25 v25.5,4.25
PA16_S1_MOSI  (via drill 0.2)
  Top 0.19: v22.75,17 22.75,15.25 U1.25
  PWR 0.19: 50,22.62 J5.3
  Bottom 0.19: 31,20.38 30.75,20.15
  Bottom 0.2: 31,20.38 45.08,20.38 46.1,21.4 48.81,21.4 J5.3 | 30.75,20.15 26.85,20.15 26.2,20.8 23,20.8 22.4,20.2 22.4,17.35 v22.75,17
PA17_S1_SCK  (via drill 0.2)
  Top 0.19: U1.26 22.3,14.75 22,15.05 22,17.25 22.88,18.12 22.88,18.75 22.05,19.57 19.75,19.57 19.25,20.07 19.25,21.12 v19.5,21.38
  MID 0.19: v19.5,21.38 21.12,23 21.12,23.12 21.88,23.88 46.38,23.88 47.5,22.75 J5.4
PA18_OTG  (via drill 0.2)
  Top 0.19: U1.27 22.3,14.25 21.62,14.93 21.62,15.38 21,16 17,16 14.5,13.5 v8.88,13.5
  Top 0.2: J1.4 4.89,11.86 v4.85,11.85 | R21.2 v7.65,16.95 7.45,16.75 Q3.G 7.95,15.72 v7.95,15.45
  Bottom 0.19: 4.82,11.82 v4.85,11.85
  Bottom 0.2: v4.85,11.85 4.9,11.85 4.9,12.74 4.9,15.05 6.8,16.95 v7.65,16.95 | 8.9,13.5 v8.88,13.5 8.95,13.5 9.15,13.7 9.15,14.25 v7.95,15.45
PA19_S1_MISO  (via drill 0.2)
  Top 0.2: U1.28 21.55,13.75 v21.3,14
  PWR 0.2: v21.3,14 26.55,14 30.7,18.15 30.7,18.6 30.4,18.9 30.4,20.4 31.25,21.27 33.08,21.27 v33.6,21.8
  MID 0.2: v33.6,21.8 33.6,21.6 33.8,21.5 43.84,21.5 J5.5
PA20_TCC0-W6  (via drill 0.2)
  Top 0.2: Q1.G 15.32,22.73 R16.2 15.25,22.65 v14.5,22.65 | 20.8,15.4 v20.8,15.5 21.1,15.2 21.1,14.65 20.85,14.4 20.85,13.6 21.05,13.4 21.6,13.4 21.75,13.25 U1.29
  PWR 0.19: J5.1 55.12,22.75 53.25,24.62 16.5,24.62 14.5,22.62 v14.5,22.65
  Bottom 0.2: v20.8,15.5 20.8,17.25 R16.2 14.6,22.75 v14.5,22.65
PA21_TCC0-W7  (via drill 0.2)
  Top 0.2: J4.2 10.5,20.7 v10.8,21 | U1.30 21.75,12.75 21.5,13 20.9,13 20.5,13.4 20.5,14.7 v20.6,14.8
  MID 0.19: J5.2 52.5,22.75 51,24.25 21.12,24.25 18.12,21.25 11.12,21.25 10.88,21 v10.8,21
  Bottom 0.2: v10.8,21 11.3,21.5 11.58,21.5 EWK.X 12.48,22.4 14,22.4 14.2,22.2 15.2,22.2 20.3,17.1 20.3,15.1 v20.6,14.8
PA22_TC4-W0  (via drill 0.2)
  Top 0.19: U1.31 21.62,12.25 v21.38,12.5
  MID 0.19: v21.38,12.5 20.5,11.62 20.5,2.5 21.75,1.25 41.38,1.25 42.38,2.25 J3.9
PA23_TC4-W1  (via drill 0.2)
  Top 0.19: U1.32 21.5,11.75 v21.38,11.88
  MID 0.19: v21.38,11.88 21.88,12.38 21.88,12.62 21.5,13 21.25,13 20.12,11.88 20.12,2.38 21.62,0.88 43.5,0.88 44.88,2.25 J3.10
PA27_GPIO0  (via drill 0.2)
  Top 0.2: U1.39 24.45,7.45 v23.69,6.69 | U2.27 43.7,13.5 43.35,13.85 v43.35,14.4 | 43.3,14.45 v43.35,14.4 | v41.8,15.7 42.05,15.7 v43.35,14.4
  PWR 0.2: v19.45,4.35 23.7,4.35 24.35,3.7 33.95,3.7 41.5,11.25 41.5,15.4 v41.8,15.7 | 43.3,14.45 v43.35,14.4
  Bottom 0.2: v23.69,6.69 22.7,5.7 19.3,5.7 19,5.4 19,4.8 v19.45,4.35 | GPIO0.X 45.46,16.51 v43.35,14.4
PA28_ACK  (via drill 0.2)
  Top 0.19: U1.41 25.45,8.18 v25.55,8.07
  Top 0.2: v52,9.3 U2.7
  PWR 0.19: v25.55,8.07 25.9,7.72 25.9,7.12 | 27.02,6 27.73,6 27.75,6.03 28.4,6.03 29,6.62 v30.6,6.62
  PWR 0.2: 25.9,7.12 25.9,7 26.9,6 27.02,6
  Bottom 0.2: v30.6,6.62 33.33,6.62 34.85,8.15 51.45,8.15 52,8.7 v52,9.3
PA30_SWCLK  (via drill 0.2)
  Top 0.19: 27.27,7.5 27.45,7.67 U1.45
  Top 0.2: R4.1 24.95,20.55 24.7,20.3 v23.6,20.3 | 27.27,7.5 v27,7.5 | v42.3,8.8 R12.1
  MID 0.2: v36.5,12.5 37.6,12.5 41.3,8.8 v42.3,8.8
  Bottom 0.2: v23.6,20.3 23.6,19.1 23.1,18.6 23.1,18 24.8,16.3 24.8,14.77 J2.4 26.4,13.17 26.4,7.9 26.8,7.5 v27,7.5 27.55,6.95 28.35,6.95 29.1,7.7 29.1,11.1 30.35,12.35 36.35,12.35 v36.5,12.5
PA31_SWDIO  (via drill 0.2)
  Top 0.2: U1.46 27.95,7.95 v28,7.95 28.45,7.5 v28.45,4.85 | v42.25,10.15 R22.1
  PWR 0.2: v36.3,8.85 35.9,8.85 32.05,5 28.6,5 v28.45,4.85
  Bottom 0.2: J2.2 28.25,13.86 28.25,8.2 v28,7.95 | v36.3,8.85 37.6,10.15 v42.25,10.15
PB02_AIN10
  Top 0.2: J3.3 27.21,2.56 28.95,4.3 28.95,7.65 28.45,8.15 U1.47
PB03_AIN11
  Top 0.2: U1.48 28.95,8.45 29.3,8.1 29.3,2.79 J3.4
PB08_RST  (via drill 0.2)
  Top 0.2: U1.7 30.45,12.75 v30.6,12.9 | Q5.2 v40.7,17.3 R10.1
  Bottom 0.2: v30.6,12.9 30.7,13 32.2,13 36.5,17.3 v40.7,17.3
PB10_TCC0-W4  (via drill 0.2)
  Top 0.19: 26,16.07 U1.19
  Top 0.2: 26,16.07 26,16.75 v25.85,16.9
  MID 0.19: 33.7,15.1 31.9,16.9 29.4,16.9 28.2,18.1 27.2,18.1
  MID 0.2: 33.7,15.1 35.1,13.7 35.1,6 35.2,5.9 49.05,5.9 J3.13 | 27.2,18.1 27.05,18.1 v25.85,16.9
PB11_TCC0-W5  (via drill 0.2)
  Top 0.19: v25.4,17.5 25.4,16.07 U1.20
  MID 0.19: 29.6,17.3 28.4,18.5 26.4,18.5 v25.4,17.5
  MID 0.2: J3.14 51.2,6.3 35.6,6.3 35.5,6.4 35.5,13.8 32,17.3 29.6,17.3
PB22_S5_TX  (via drill 0.2)
  Top 0.2: U1.37 23.45,8.35 23.4,8.3 v23.4,8 | v47.55,20.2 47.55,19.5 v46.85,18.8 48,17.65 U2.23
  PWR 0.19: 32.1,9.2 30.1,9.2 29.8,9.5 23.98,9.5 U1.37 23.45,8.05 v23.4,8
  PWR 0.2: 34.8,22.62 J5.9 34.7,22.52 34.7,20.8 32.7,18.8 32.7,9.8 32.1,9.2 | v47.55,20.2 38.05,20.2 v37.4,20.85
  Bottom 0.2: v37.4,20.85 36.65,20.85 J5.9 | RXD.X 46.73,18.68 v46.85,18.8
PB23_S5_RX  (via drill 0.2)
  Top 0.2: U1.38 23.95,8.05 v24,8 | U2.22 49,17.15 48.55,17.6 48.55,19.5 v48.35,19.7
  PWR 0.19: 32.3,8.8 29.9,8.8 29.57,9.12 24.12,9.12 24,9 v24,8
  PWR 0.2: 32.3,8.8 33.1,9.6 33.1,18.39 J5.8 37.38,22.1 38.73,20.75 47.8,20.75 48.35,20.2 v48.35,19.7
  Bottom 0.2: TXD.X 48.02,16.65 47.95,16.65 47.4,17.2 47.4,18.4 47.3,18.5 47.3,19.7 47.1,19.9 47.1,20.5 47.3,20.7 47.85,20.7 48.35,20.2 v48.35,19.7
PMICINT  (via drill 0.2)
  Top 0.2: v7.7,8.7 7.65,8.75 7.65,9.1 R24.2 | U5.7 5,5.9 4.5,5.4 v3.9,5.4
  Bottom 0.19: 7.75,8.75 v7.7,8.7
  Bottom 0.2: v7.7,8.7 8.3,8.1 8.3,7.5 8,7.2 6.3,7.2 4.4,5.3 4,5.3 v3.9,5.4
RESET#
  Top 0.2: 32.34,22.62 32.34,21.55 R6.2 31.49,20.45 33,20.45 34.9,18.55 34.9,17.8 36.75,15.95 40.15,15.95 40.75,16.55 Q5.3
  Top 0.305: 32.34,22.62 J5.10
RESETN  (via drill 0.2)
  Top 0.2: R6.1 R3.2 C2.1 v29.7,19.6 R5.1 | U1.40 24.95,7.75 v25.35,7.35 | R2.2 20.2,8.9 19.7,8.4 19.2,8.4 18.9,8.1 18.9,5.8 v19.5,5.2
  MID 0.2: v29.7,19.6 29,18.9 26.1,18.9 24.9,17.7 24.9,7.8 v25.35,7.35
  Bottom 0.2: v19.5,5.2 23.2,5.2 v25.35,7.35
STAT  (via drill 0.2)
  Top 0.305: U5.4 7.65,7.65 v7.7,7.7 | 3,6.1 DL2.C 3,6 v4.2,6
  Bottom 0.305: v7.7,7.7 5.9,7.7 v4.2,6
USB_N  (via drill 0.2)
  Top 0.19: J1.2 arc90 4.29,12.98 7.9,12.98 | U1.33 21.58,11.25 arc-90 20.93,11.9 20.93,11.85 arc90 19.8,12.98 7.9,12.98 | 7.9,12.98 8,13.08 8,13.8
  Top 0.24: v8,14.7 D1.3 D-.X 8,13.8
  Bottom 0.19: 8.2,14 D-.X
  Bottom 0.24: v8,14.7 8,14.1 D-.X
USB_P  (via drill 0.2)
  Top 0.19: J1.3 arc-90 4.24,12.62 7.9,12.62 | U1.34 21.72,10.75 arc-90 20.57,11.8 20.57,11.85 arc90 19.8,12.62 7.9,12.62 | D1.2 8,12.52 7.9,12.62
  Top 0.24: D1.2 v8,10.9
  Bottom 0.24: 8,11.5 D+.X 8,11.6 v8,10.9
VBATT  (via drill 0.2)
  Top 0.2: R8.2 40,4.5 v40.1,4.4
  Top 0.305: U5.14 U5.13
  Top 0.61: U5.13 v6.5,2.5 | v14.1,10.1 14.1,11.25 D2.C 12.2,11.3 F2.2
  PWR 0.2: v6.5,2.5 U5.13 6.8,2.65 9.45,2.65 9.9,3.1 14.4,3.1 v15.8,1.7
  Bottom 0.2: v40.1,4.4 40.1,4 39.8,3.7 17.8,3.7 v15.8,1.7
  Bottom 0.61: v6.5,2.5 8.85,2.5 9.88,3.5 13,3.5 14.1,4.6 BATT+.X v14.1,10.1
VIN  (via drill 0.2)
  Top 0.2: Q2.A 10.65,11.1 | R19.2 10.65,11.1 | 10.65,11.1 v10.6,11.35 | Q2.G 10,8.4 v9.8,8.2
  PWR 0.2: v9.8,8.2 10.1,8.5 10.1,10.65 v10.6,11.35
  PWR 0.61: v10.6,11.35 10.6,17.5 12.7,19.6 21.61,19.6 J5.13 24.7,22.64
VUSB1  (via drill 0.2)
  Top 0.305: U5.23 10.5,5.4 10.8,5.7 v11,5.7
  Top 0.61: v13.9,21.7 D3.A | v12.7,14.4 12.6,14.3 C12.1 11.2,15.1 C13.1
  Bottom 0.61: v11,5.7 12.2,5.7 12.7,6.2 v12.7,14.4 12.7,20.5 v13.9,21.7

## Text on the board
test-probe: 5V | VIN(5V) | VCC | GND | RESET | 14 | 13 | 12 | 11 | 10 | 9 | 8 | 7 | 6 | USB_5V | USB_D- | SWCLK | SWDIO | JGND | JRST | VTG | BATT+ | BATT- | USB_D+ | USB_GND | AREF | A0 | A1 | A2 | A3 | A4 | A5 | A6 | 0 | 1 | 2 | 3 | 4 | 5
